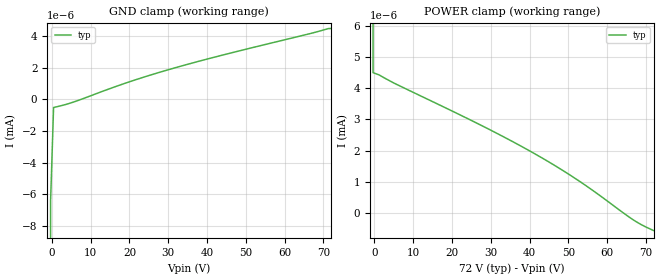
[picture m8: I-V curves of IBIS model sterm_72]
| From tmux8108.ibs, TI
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| sterm_72
[Model]   sterm_72
Model_type   Terminator
|   typ   min   max
C_comp   4.014581e-12   NA   NA
[Voltage Range]   72   NA   NA
[Temperature Range]   27   NA   NA
[Power Clamp Reference]   72   NA   NA
[GND Clamp Reference]   0   NA   NA
[GND Clamp]
|   Voltage   I(typ)   I(min)   I(max)
-5V       -1.144A    NA         NA
-1.111V   -36.36mA   NA         NA
-333.3mV  -6.477nA   NA         NA
444.4mV   -524.1pA   NA         NA
5.111V    -218.2pA   NA         NA
19.11V    1.024nA    NA         NA
31.56V    1.967nA    NA         NA
46.33V    2.929nA    NA         NA
72V       4.464nA    NA         NA
[POWER Clamp]
|   Voltage   I(typ)   I(min)   I(max)
-5V       744mA      NA         NA
-1.111V   26.13mA    NA         NA
-333.3mV  4.496nA    NA         NA
1.222V    4.424nA    NA         NA
5.111V    4.16nA     NA         NA
26.89V    2.853nA    NA         NA
40.89V    1.936nA    NA         NA
52.56V    1.052nA    NA         NA
66.56V    -191.2pA   NA         NA
68.89V    -365.1pA   NA         NA
72V       -549pA     NA         NA
